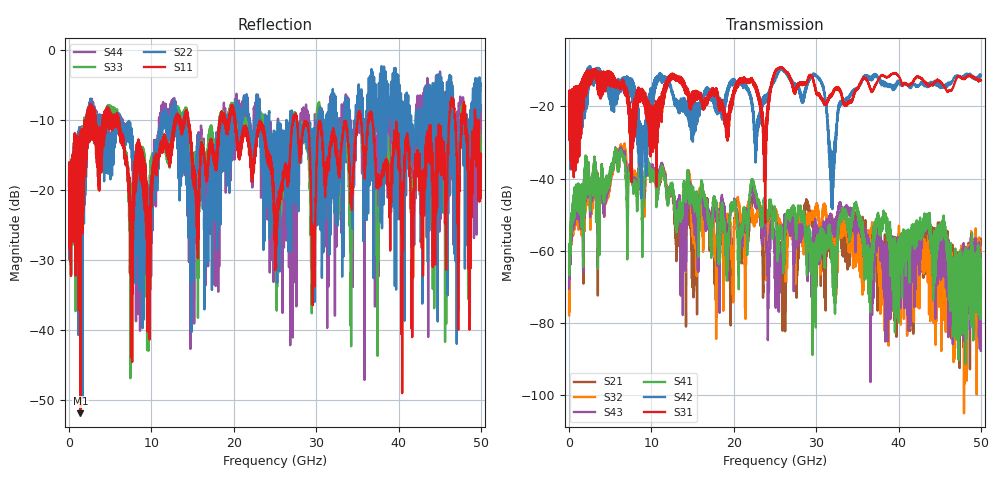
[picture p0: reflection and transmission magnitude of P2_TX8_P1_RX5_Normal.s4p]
!Keysight Technologies,N5225B,MY57041031,A.13.20.10
!Date: Friday, May 31, 2019 11:22:04
!Correction: S11(Full 4 Port(1,2,3,4))
!S12(Full 4 Port(1,2,3,4))
!S13(Full 4 Port(1,2,3,4))
!S14(Full 4 Port(1,2,3,4))
!S21(Full 4 Port(1,2,3,4))
!S22(Full 4 Port(1,2,3,4))
!S23(Full 4 Port(1,2,3,4))
!S24(Full 4 Port(1,2,3,4))
!S31(Full 4 Port(1,2,3,4))
!S32(Full 4 Port(1,2,3,4))
!S33(Full 4 Port(1,2,3,4))
!S34(Full 4 Port(1,2,3,4))
!S41(Full 4 Port(1,2,3,4))
!S42(Full 4 Port(1,2,3,4))
!S43(Full 4 Port(1,2,3,4))
!S44(Full 4 Port(1,2,3,4))
!S4P File: Measurements: <S11,S12,S13,S14>,
!<S21,S22,S23,S24>,
!<S31,S32,S33,S34>,
!<S41,S42,S43,S44>:
# Hz S  dB  R 50.0
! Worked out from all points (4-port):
!   5000 points, 10 MHz to 50 GHz, reference 50 ohm
!   strongest paths, dB at 10 MHz, 12.51 GHz, 25.01 GHz, 37.51 GHz, 50 GHz:
!     S31: -19.4, -11.5, -10.3, -12.8, -12.8
!     S42: -19.4, -15.6, -12.9, -11.8, -11.4
!     S41: -58.2, -41.1, -50.1, -49.5, -67.0
!     S43: -70.5, -41.6, -61.5, -53.2, -87.7
!     S32: -77.9, -41.7, -49.5, -56.5, -72.7
!     S21: -64.2, -42.5, -50.2, -62.1, -62.7
!   lowest |S11| = -52.0 dB at 1.38 GHz (marker M1), VSWR 1.01, Z = 49.9 - j0.22 ohm
!   |S11| at or under -10 dB: 20.17 GHz to 27.18 GHz (7.013 GHz wide, 29.6 % of centre); 27.67 GHz to 35.04 GHz (7.368 GHz wide, 23.5 % of centre); 36.79 GHz to 46.16 GHz (9.374 GHz wide, 22.6 % of centre)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
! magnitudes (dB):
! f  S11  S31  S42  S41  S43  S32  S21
! 10 MHz  -19.5  -19.4  -19.4  -58.2  -70.5  -77.9  -64.2
! 1.38 GHz  -52.0  -28.8  -25.8  -44.1  -45.6  -45.2  -44.5
! 22.27 GHz  -16.4  -12.6  -19.4  -40.3  -41.7  -48.6  -45.3
! 29.84 GHz  -33.6  -14.4  -11.2  -76.0  -54.1  -50.5  -56.0
! 31.94 GHz  -11.7  -16.4  -35.6  -61.1  -52.1  -51.2  -52.9
! 35.92 GHz  -17.4  -12.1  -11.4  -59.8  -54.4  -60.5  -55.0
! 50 GHz  -14.9  -12.8  -11.4  -67.0  -87.7  -72.7  -62.7
